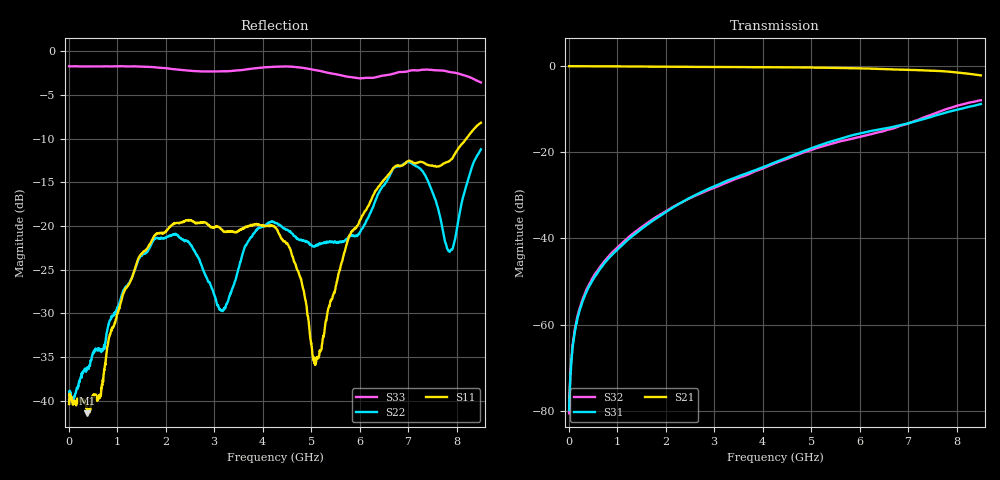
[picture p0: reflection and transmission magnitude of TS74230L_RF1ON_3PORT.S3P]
!Agilent Technologies,E5071C,MY46522130,B.12.04
!Date: Fri Aug 01 10:37:56 2025
!Data & Calibration Information:
!Freq	S11:SOLT3(ON)	S13:SOLT3(ON)	S14:SOLT3(ON)
!	S31:SOLT3(ON)	S33:SOLT3(ON)	S34:SOLT3(ON)
!	S41:SOLT3(ON)	S43:SOLT3(ON)	S44:SOLT3(ON)
!PortZ  Port1:50+j0  Port3:50+j0  Port4:50+j0
!Above PortZ is port z conversion or system Z0 setting when saving the data.
!When reading, reference impedance value at option line is always used.
# Hz S dB R 50
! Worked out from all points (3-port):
!   1601 points, 10 MHz to 8.5 GHz, reference 50 ohm
!   strongest paths, dB at 10 MHz, 2.132 GHz, 4.255 GHz, 6.378 GHz, 8.5 GHz:
!     S21: -0.1, -0.3, -0.4, -0.8, -2.3
!     S31: -79.8, -33.0, -22.4, -14.8, -8.9
!     S32: -80.5, -32.8, -22.6, -15.5, -8.0
!   lowest |S11| = -41.5 dB at 381.4 MHz (marker M1), VSWR 1.02, Z = 50.6 - j0.583 ohm
!   |S11| at or under -10 dB: start of sweep to 8.197 GHz
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1e7  -40.40 19.3  -0.13 -0.4  -80.68 23.9
     -0.13 -0.4  -40.37 18.1  -79.12 35.0
     -79.75 31.4  -80.50 45.2  -1.71 179.4
1.320438e8  -40.06 -12.5  -0.14 -2.6  -61.34 85.1
            -0.14 -2.7  -39.36 -11.4  -60.92 85.1
            -61.28 85.0  -60.71 83.3  -1.72 176.7
3.814375e8  -41.46 -42.9  -0.15 -7.5  -52.05 93.4
            -0.16 -7.6  -36.43 -28.5  -51.59 90.5
            -52.06 92.7  -51.59 90.8  -1.74 170.9
1.787594e9  -21.06 -115.7  -0.24 -35.2  -35.55 100.9
            -0.25 -35.2  -21.42 -127.6  -35.20 91.0
            -35.52 100.8  -35.16 90.9  -1.84 141.9
3.156606e9  -20.41 -62.2  -0.31 -62.4  -27.23 85.6
            -0.32 -62.4  -29.70 112.6  -27.55 73.0
            -27.20 85.4  -27.58 72.9  -2.29 100.3
4.255e9  -20.16 0.0  -0.38 -85.6  -22.35 69.5
         -0.39 -85.7  -19.65 18.2  -22.65 56.1
         -22.39 69.2  -22.63 56.0  -1.78 72.7
5.109306e9  -35.26 -51.1  -0.46 -104.8  -18.69 51.4
            -0.47 -104.9  -22.17 53.5  -19.12 36.6
            -18.69 51.5  -19.12 36.8  -2.18 54.4
6.350969e9  -15.85 -76.8  -0.73 -135.2  -14.83 17.2
            -0.74 -135.3  -16.77 -30.3  -15.57 6.9
            -14.89 17.4  -15.52 6.9  -2.94 1.2
7.873862e9  -12.45 6.5  -1.44 -179.3  -10.64 -23.7
            -1.45 -179.5  -22.81 -14.0  -9.73 -34.4
            -10.58 -23.2  -9.79 -34.2  -2.39 -23.7
8.5e9  -8.19 37.6  -2.26 158.8  -8.89 -47.3
       -2.27 158.6  -11.24 33.9  -8.11 -62.4
       -8.90 -47.2  -8.02 -62.4  -3.57 -31.6
